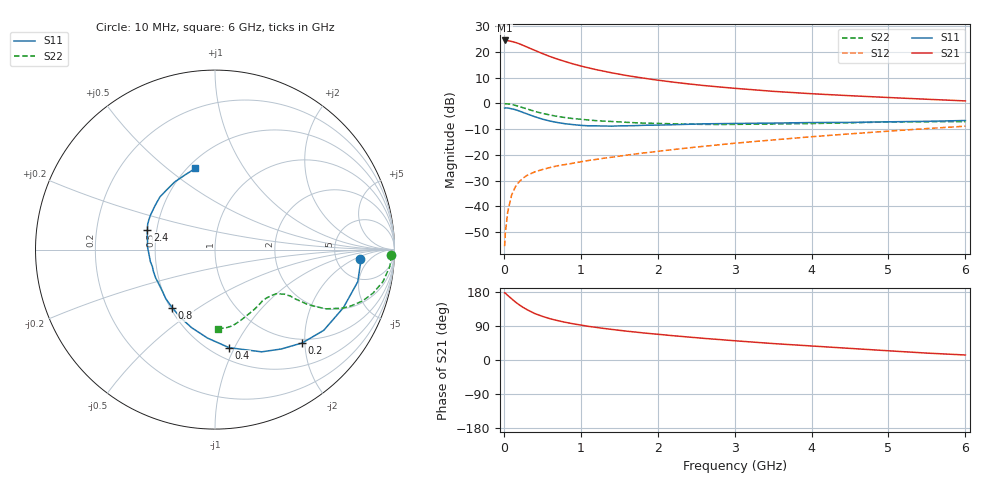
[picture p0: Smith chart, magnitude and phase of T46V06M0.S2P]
! Infineon Technologies  Discrete & RF Semiconductors
! BFR182T
! Si NPN RF Bipolar Junction Transistor in SC75
! VCE = 6 V  IC = 6 mA
! Common Emitter S-Parameters:  October  1999
# GHz  S  MA  R  50
!  f  S11  S21  S12  S22
! GHz  MAG  ANG  MAG  ANG  MAG  ANG  MAG  ANG
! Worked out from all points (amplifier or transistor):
!   36 points, 10 MHz to 6 GHz, reference 50 ohm
!   highest |S21| = 24.4 dB at 10 MHz (marker M1)
!   |S21| within 3 dB of that: start of sweep to 336 MHz
!   unconditionally stable (mu >= 1): 1.354 GHz to 4.035 GHz
!   at 250 MHz: K = 0.32, MSG = 25.8 dB, |S12| = -29.0 dB
!   at 1.4 GHz: K = 1.02, MAG = 15.6 dB, |S12| = -20.9 dB
!   at 6 GHz: K = 0.85, MSG = 4.9 dB, |S12| = -8.8 dB
!   lowest NFmin = 1.25 dB at 450 MHz
!   S11 on the Smith chart (normalised r, x): 10 MHz: 8.83, -2.64; 200 MHz: 0.92, -1.95; 400 MHz: 0.61, -0.95; 800 MHz: 0.51, -0.40; 2.4 GHz: 0.44, +0.12; 6 GHz: 0.55, +0.63
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0.01  0.8119 -3.6  16.6 177.1  0.0017 72.9  0.981 -1.9
0.02  0.816 -3.7  16.49 176.3  0.0031 108.5  0.9828 -2.2
0.05  0.8153 -12.7  16.48 170.5  0.0078 87.4  0.9781 -5.6
0.1  0.785 -24.4  15.89 161.8  0.0165 79.0  0.9528 -10.8
0.15  0.7545 -36.6  15.19 153.1  0.0241 72.3  0.9133 -15.4
0.2  0.712 -46.9  14.33 145.6  0.0303 69.0  0.8705 -19.2
0.25  0.6656 -56.3  13.35 138.9  0.0355 64.2  0.823 -22.3
0.3  0.626 -65.5  12.39 133.0  0.04 62.0  0.7809 -24.7
0.4  0.552 -81.8  10.7 122.8  0.0468 57.9  0.7007 -28.1
0.5  0.4949 -94.8  9.265 115.3  0.0521 55.6  0.6411 -29.6
0.6  0.4537 -106.8  8.106 108.9  0.057 54.5  0.5947 -30.7
0.7  0.4244 -117.0  7.198 103.9  0.0617 54.4  0.5572 -31.1
0.8  0.402 -126.3  6.453 99.4  0.0653 54.9  0.5296 -31.5
1.1  0.3668 -148.8  4.884 88.8  0.0781 56.3  0.4754 -32.3
1.4  0.3615 -165.1  3.918 80.8  0.0901 58.1  0.445 -33.8
1.6  0.3676 -174.1  3.462 76.0  0.0993 59.1  0.4286 -34.8
2.2  0.3852 168.2  2.583 64.1  0.127 61.4  0.4019 -40.4
2.4  0.3929 163.6  2.385 60.6  0.137 62.0  0.3949 -42.7
3.5  0.4146 143.5  1.712 43.4  0.1954 61.4  0.3983 -56.3
4.5  0.4279 129.1  1.408 30.6  0.2564 58.5  0.4197 -70.1
5.5  0.4485 111.8  1.202 18.2  0.3246 53.9  0.4406 -82.6
6  0.4652 103.7  1.116 13.2  0.361 50.7  0.4402 -87.8
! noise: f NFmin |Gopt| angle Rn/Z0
0.45  1.25  0.25  39  0.3
0.9  1.4  0.25  78  0.23
1.8  1.95  0.21  151  0.2
